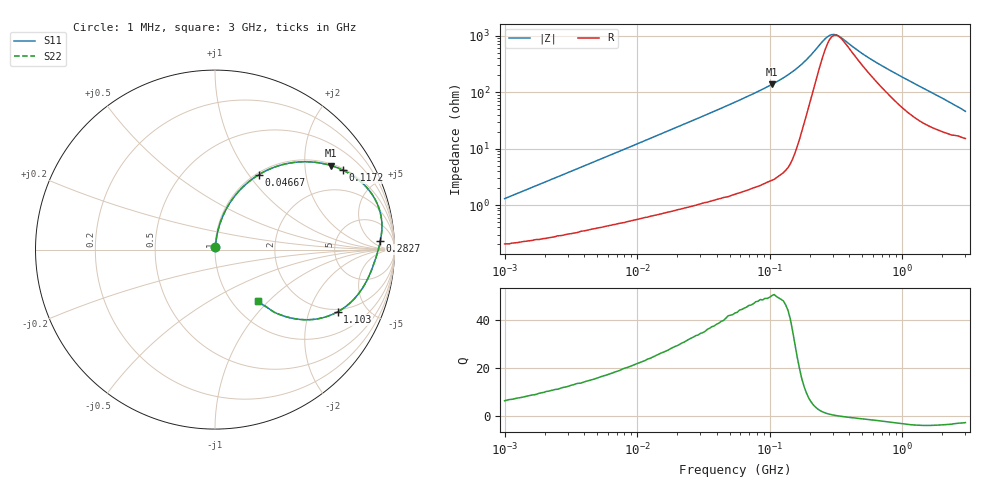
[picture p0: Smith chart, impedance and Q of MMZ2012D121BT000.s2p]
! S-parameter Generated by TDK Corporation
! Copyright(C) 2016 TDK Corporation.
! All Rights Reserved.
! TDK P/N: MMZ2012D121BT000 (Chip Beads)
! Property: |Z|=120¶ at 100MHz
! Size(LxWxT): 2x1.25x0.85mm, 0.079x0.049x0.033inches
! Model Type: s2p (Touchstone File Format Version 1.0)
! Frequency: DC=Yes Start=1MHz Stop=3000MHz 202points Log-sweep
! Note: This model was converted from impedance.
! Model Generated on May. 16, 2016
! Hash(MD5):
! Port Assignments:
!  1 ---@@@--- 2
! Applicable Conditions:
!  Temperature = 25 degC
!  DC Bias Current = 0 A
!  Small Signal Operation
! Terms and conditions regarding TDK Simulation Models
! (1)This simulation model is being provided solely for informational purposes. Please refer to the specifications of the products in terms of detailed characteristics of such products.
! (2)In no event shall TDK Corporation of any of its subsidiaries be liable for any loss or damage arising, directly or indirectly,
!  From any information contained in this simulation model, including, but not limited to loss or damages arising from any inaccuracies, omissions or errors in connection with such information.
! (3)Any and all copyrights on this simulation model are owned by TDK Corporation.
!  Duplication or redistribution of this simulation model without prior written permission from TDK Corporation is prohibited.
! (4)This simulation model is subject to any modification or change without any prior notice.
! (5)Neither TDK Corporation nor any of its subsidiaries shall make any warranty, express or implied,
!  Including but not limited to the correctness, implied warranties of merchantability and fitness for a particular purpose with respect to this simulation models.
! (6)The use of this simulation model shall be deemed to have consented to the terms and conditions hereof.
# MHz S MA R 50
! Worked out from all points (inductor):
!   201 points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, 1 MHz to 3 GHz, reference 50 ohm
!   read as one part in series: L = 203 nH near 1.041 MHz
!   highest Q = 49.7 at 103.9 MHz (marker M1), where L = 209 nH
!   self-resonance near 323.9 MHz
!   S11 on the Smith chart (normalised r, x): 1 MHz: 1.00, +0.03; 46.67 MHz: 1.03, +1.12; 117.2 MHz: 1.07, +3.20; 282.7 MHz: 18, +11; 1.103 GHz: 1.87, -3.15; 3 GHz: 1.30, -0.86
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1  0.01296 80.2  0.9979 -0.7  0.9979 -0.7  0.01296 80.2
3.900413  0.04807 83.1  0.9954 -2.7  0.9954 -2.7  0.04807 83.1
8.017732  0.09642 81.6  0.9905 -5.5  0.9905 -5.5  0.09642 81.6
14.61624  0.1717 77.9  0.9785 -9.9  0.9785 -9.9  0.1717 77.9
27.73354  0.3115 70.1  0.941 -18.1  0.941 -18.1  0.3115 70.1
46.66789  0.4843 59.6  0.8631 -29.0  0.8631 -29.0  0.4843 59.6
54.77226  0.5468 55.5  0.8246 -33.1  0.8246 -33.1  0.5468 55.5
78.52918  0.6927 45.0  0.7068 -43.8  0.7068 -43.8  0.6927 45.0
103.9275  0.7993 35.8  0.5851 -53.1  0.5851 -53.1  0.7993 35.8
117.1891  0.8401 31.7  0.5256 -57.1  0.5256 -57.1  0.8401 31.7
161.4254  0.9238 20.3  0.347 -67.4  0.347 -67.4  0.9238 20.3
213.6344  0.9431 10.5  0.1864 -67.1  0.1864 -67.1  0.9431 10.5
260.9752  0.9294 4.8  0.1069 -46.3  0.1069 -46.3  0.9294 4.8
282.7291  0.9219 2.9  0.09165 -30.2  0.09165 -30.2  0.9219 2.9
306.2963  0.9147 1.1  0.0873 -11.8  0.0873 -11.8  0.9147 1.1
331.8279  0.9078 -0.5  0.09262 5.0  0.09262 5.0  0.9078 -0.5
515.4121  0.8742 -8.8  0.1911 44.5  0.1911 44.5  0.8742 -8.8
800.5644  0.8294 -18.4  0.3371 50.8  0.3371 50.8  0.8294 -18.4
1102.76  0.7666 -26.9  0.4693 47.6  0.4693 47.6  0.7666 -26.9
1402.151  0.6933 -33.7  0.572 42.3  0.572 42.3  0.6933 -33.7
1782.824  0.6008 -40.2  0.6653 35.6  0.6653 35.6  0.6008 -40.2
3000  0.3712 -50.2  0.814 20.5  0.814 20.5  0.3712 -50.2
